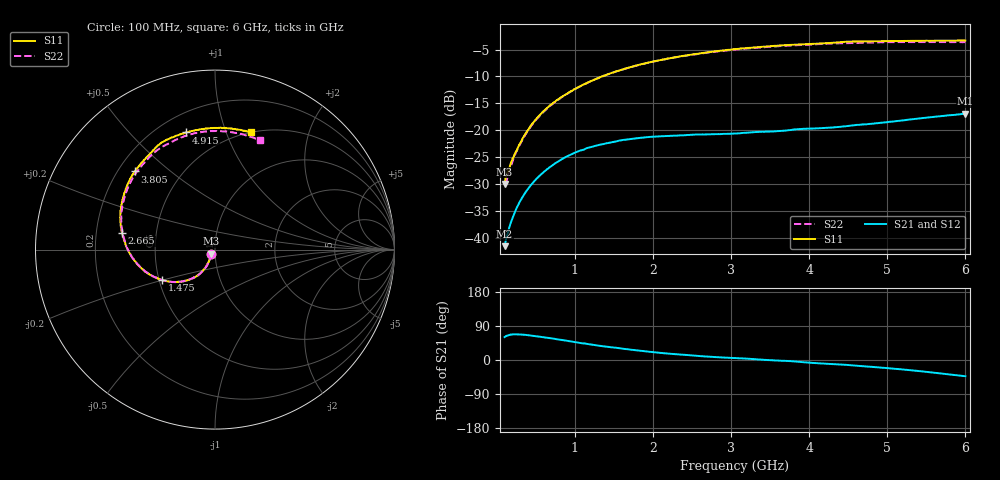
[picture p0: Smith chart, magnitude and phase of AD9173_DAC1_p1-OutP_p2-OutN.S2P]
! Created Thu Dec 01 15:07:18 2016
# mhz S ma R 50
! 2 Port Network Data from Sweep1.SP1.SP block
! freq  magS11  angS11  magS21  angS21  magS12  angS12  magS22  angS22
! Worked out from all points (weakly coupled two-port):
!   1181 points, 100 MHz to 6 GHz, reference 50 ohm
!   highest |S21| = -16.92 dB at 6 GHz (marker M1); lowest = -41.6 dB at 100 MHz (marker M2)
!   lowest |S11| = -30.0 dB at 100 MHz (marker M3), VSWR 1.07, Z = 47.9 - j2.25 ohm
!   |S11| at or under -10 dB: start of sweep to 1.35 GHz
!   |S22| runs from -30.0 to -3.6 dB; largest |S21 - S12| = 0.0005
!   S11 on the Smith chart (normalised r, x): 100 MHz: 0.96, -0.05; 1.475 GHz: 0.52, -0.20; 2.665 GHz: 0.31, +0.08; 3.805 GHz: 0.27, +0.38; 4.915 GHz: 0.31, +0.73; 6 GHz: 0.50, +1.22
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100  0.03157 -132.0  0.008316 60.6  0.008402 60.3  0.03146 -135.7
125  0.03874 -128.0  0.01012 64.1  0.009997 63.6  0.03394 -129.9
175  0.04796 -122.2  0.01344 66.9  0.01342 66.7  0.04511 -122.4
250  0.06362 -118.5  0.0185 67.7  0.01848 67.6  0.06334 -117.4
330  0.08278 -117.3  0.02387 66.9  0.02389 66.7  0.08227 -116.1
435  0.1101 -118.2  0.03074 64.5  0.03069 64.5  0.1078 -117.1
565  0.1417 -120.6  0.03878 61.2  0.0386 61.0  0.1398 -120.0
700  0.1743 -124.1  0.04641 57.1  0.04633 57.0  0.1722 -123.7
880  0.2139 -129.8  0.05609 51.5  0.05602 51.4  0.2124 -129.7
1085  0.2603 -136.2  0.06498 44.4  0.06497 44.4  0.2599 -136.7
1475  0.3417 -150.2  0.07719 33.5  0.07703 33.6  0.3403 -150.2
2070  0.4447 -170.5  0.08743 19.2  0.08756 19.3  0.4452 -170.6
2665  0.525 169.9  0.09126 9.3  0.0912 9.4  0.5223 169.9
3050  0.5666 158.1  0.09313 5.0  0.09294 5.0  0.5622 157.7
3465  0.6021 145.7  0.09694 -0.1  0.09688 -0.1  0.5939 144.9
3805  0.6237 135.7  0.1014 -3.7  0.1015 -3.8  0.6149 134.6
4035  0.635 129.3  0.1035 -7.6  0.1033 -7.6  0.627 127.9
4555  0.668 114.2  0.1105 -14.2  0.1104 -14.2  0.6459 112.2
4915  0.6725 104.0  0.1169 -20.1  0.117 -20.1  0.6566 101.6
5020  0.6733 101.1  0.1192 -21.8  0.1193 -21.9  0.6587 98.4
5500  0.6798 87.4  0.1306 -31.3  0.1306 -31.3  0.6597 83.5
6000  0.6831 73.1  0.1425 -42.9  0.1424 -43.0  0.6585 67.5
